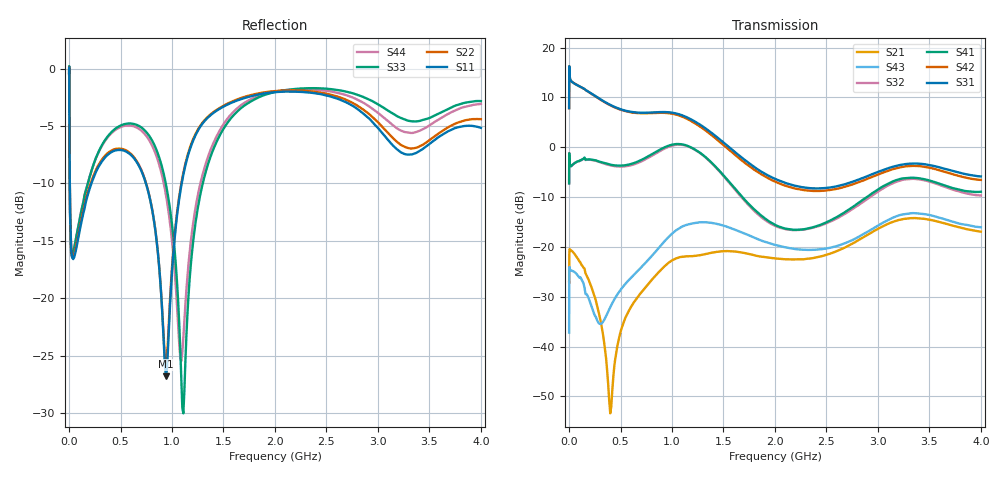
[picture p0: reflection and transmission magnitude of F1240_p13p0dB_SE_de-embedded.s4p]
! Integrated Device Technology
! Corporate Headquarters
! 6024 Silver Creek Valley Road
! San Jose, CA 95138  USA
! Phone:  1-408-284-8200
! Toll Free:  1-800-223-1366
! Webpage:  http://www.idt.com/
! Timing and RF Division
! 515 Groton Road, Suite 102
! Westford, MA 01886-6024
! Device:  F1240
! Description: Dual Intermediate Frequency Digital Variable Gain Amplifier
! Frequency:  10.0 -  500.00 MHz
! Package:  5x5 mm QFN Plastic Package: 32 pin
! Ports:  8 RF, 20 DC
!  Pin  1  = GA3 / Data  Pin 17  = RF OUT_B+
!  Pin  2  = GA4 / CLK  Pin 18  = RF OUT_B-
!  Pin  3  = GA5  Pin 19  = STBY_B
!  Pin  4  = VMODE  Pin 20  = Ground
!  Pin  5  = No Connect  Pin 21  = Ground
!  Pin  6  = GB5  Pin 22  = STB_A
!  Pin  7  = GB4  Pin 23  = RF OUT_A-  = Port 4
!  Pin  8  = GB3  Pin 24  = RF OUT_A+  = Port 3
!  Pin  9  = GB2  Pin 25  = GA0
!  Pin 10  = GB1  Pin 26  = ISET_A
!  Pin 11  = RF IN_B+  Pin 27  = VCC
!  Pin 12  = RF IN_B-  Pin 28  = Ground
!  Pin 13  = Ground  Pin 29  = RF IN_A-  = Port 2
!  Pin 14  = VCC  Pin 30  = RF IN_A+  = Port 1
!  Pin 15  = ISET_B  Pin 31  = GA1
!  Pin 16  = GB0  Pin 32  = GA2 / CSb
! Gain  = +19.5 dB
! State  = 1
! Voltage  = +5.00 V
! Current  = 85.292 mA (one channel only)
! Temperture  =  +25 C
! Test Date  =  2017-10-18
! Board  =  EB4031
! Data:  The device was measured on a custom evaluation board which has
!  individual transmission lines to the RF pins.  Data was collected
!  using a calibrated network analyzer.  The evaluation board was
!  de-embedded using Automatic Fixture Removal.
!  The reference plane is the edge of the package pin.
!  Only Channel A was measured.
!  This data is in single-ended operation.  If your needs are balanced
!  or differential S-parameters then this file needs to be used a
!  linear simulator.
! File Date:  2017-11-10  MJV
! Note:
!  Integrated Device Technology supplies this data as a sample of measured
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# Hz S dB R 100
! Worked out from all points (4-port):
!   410 points, 500 kHz to 4 GHz, reference 100 ohm
!   strongest paths, dB at 500 kHz, 930 MHz, 1.96 GHz, 2.98 GHz, 4 GHz:
!     S31: 7.8, 7.1, -6.0, -5.1, -5.9
!     S42: 7.8, 6.9, -6.5, -5.7, -6.6
!     S41: -7.3, 0.0, -15.1, -8.8, -8.9
!     S32: -7.2, -0.2, -15.4, -9.2, -9.7
!     S43: -37.2, -18.8, -19.4, -16.0, -16.1
!     S21: -27.0, -23.8, -22.2, -16.6, -16.9
!   lowest |S11| = -26.8 dB at 940 MHz (marker M1), VSWR 1.10, Z = 108 + j5.66 ohm
!   |S11| at or under -10 dB: 7.319 MHz to 217.1 MHz (209.8 MHz wide, 187 % of centre); 746.6 MHz to 1.094 GHz (347.4 MHz wide, 37.8 % of centre)
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500000  -0.37 -5.9  -27.03 -0.2  -27.29 78.5  -59.60 67.7
        -27.02 -0.6  -0.37 -5.8  -59.30 66.9  -27.28 79.7
        7.85 -105.2  -7.22 70.9  -0.46 1.2  -37.26 -136.0
        -7.25 72.1  7.83 -104.0  -37.20 -135.9  -0.47 3.5
3000000  -3.93 -56.5  -21.07 13.4  -17.84 17.8  -42.53 62.5
         -21.07 13.4  -3.90 -56.5  -42.48 62.4  -17.85 18.0
         15.62 -174.5  -2.35 -6.7  -3.49 -52.0  -24.06 47.2
         -2.33 -6.6  15.62 -174.3  -24.03 47.1  -3.55 -51.8
2e8  -10.45 -121.2  -27.03 -94.6  -20.41 -51.6  -34.15 11.4
     -27.14 -93.2  -10.24 -122.6  -34.13 11.8  -20.43 -51.6
     11.00 109.4  -2.51 -46.3  -9.43 -84.9  -30.03 -116.8
     -2.45 -46.5  10.96 108.6  -30.85 -114.9  -9.43 -84.1
5.4e8  -7.17 -176.4  -35.36 10.2  -22.02 -108.9  -28.15 -58.4
       -34.60 2.3  -7.06 -177.7  -28.30 -56.8  -22.17 -109.2
       7.37 24.8  -3.85 -116.8  -4.83 -153.5  -29.00 35.7
       -3.63 -118.1  7.28 23.8  -27.58 24.9  -4.97 -153.4
9.4e8  -26.79 35.0  -22.99 -68.6  -19.61 168.3  -23.97 -152.9
       -23.66 -78.6  -25.92 30.5  -24.28 -147.7  -19.99 167.7
       7.05 -73.3  -0.15 152.6  -10.03 142.0  -19.61 -51.9
       0.09 148.2  6.88 -75.1  -18.58 -63.7  -10.95 144.5
1.52e9  -3.21 -148.0  -20.43 149.5  -25.43 32.6  -26.01 71.8
        -20.85 153.4  -3.13 -148.0  -25.84 77.6  -26.54 31.9
        0.60 125.4  -6.26 -31.2  -4.96 -133.0  -16.20 140.0
        -6.11 -36.4  0.08 124.1  -15.86 135.0  -4.58 -136.2
4e9  -5.16 -155.0  -16.99 65.9  -21.27 -50.3  -20.05 -48.3
     -16.95 65.3  -4.40 -149.8  -22.17 -29.3  -24.34 -40.1
     -5.86 12.4  -9.68 -112.8  -2.82 -137.4  -15.75 90.2
     -8.94 -124.6  -6.56 21.5  -16.05 62.9  -3.07 -143.2
